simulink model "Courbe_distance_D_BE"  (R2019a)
settings: Solver=VariableStepAuto  StartTime=0.0  StopTime=6.283185307  MaxStep=0.001  RelTol=1e-6  SampleTimeConstraint=STIndependent

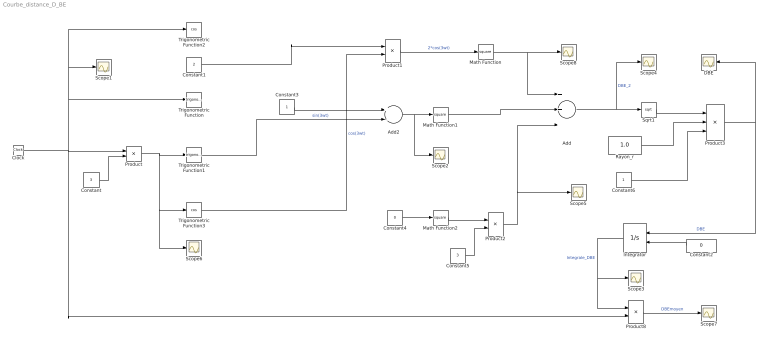
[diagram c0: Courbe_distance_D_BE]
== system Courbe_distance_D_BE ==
  Add : Sum  Inputs=+++
  Add2 : Sum  Inputs=+-
  Clock : Clock
  Constant : Constant  Value=3
  Constant1 : Constant  Value=2
  Constant2 : Constant  Value=0
  Constant3 : Constant
  Constant4 : Constant  Value=0
  Constant5 : Constant  Value=3
  Constant6 : Constant
  DBE : Scope
  Integrator : Integrator  InitialConditionSource=external
  Math Function : Math  Operator=square
  Math Function1 : Math  Operator=square
  Math Function2 : Math  Operator=square
  Product : Product
  Product1 : Product
  Product2 : Product
  Product3 : Product  Inputs=**/
  Product8 : Product  Inputs=*/
  Rayon_r : Constant  Value=1.0
  Scope{1..8} (8 alike) : Scope
  Sqrt1 : Sqrt
  Trigonometric Function : Trigonometry
  Trigonometric Function1 : Trigonometry
  Trigonometric Function2 : Trigonometry  Operator=cos
  Trigonometric Function3 : Trigonometry  Operator=cos
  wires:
  Product/1 -> Scope6/1, Trigonometric Function3/1, Trigonometric Function1/1
  Constant/1 -> Product/2
  Clock/1 -> Product8/2, Trigonometric Function/1, Trigonometric Function2/1, Scope1/1, Product/1
  Add2/1 -> Scope2/1, Math Function1/1
  Math Function/1 -> Scope8/1, Add/1
  Add/1 -> Sqrt1/1, Scope4/1  "DBE_2"
  Integrator/1 -> Product8/1, Scope3/1  "Integrale_DBE"
  Constant2/1 -> Integrator/2
  Product8/1 -> Scope7/1  "DBEmoyen"
  Trigonometric Function3/1 -> Product1/2  "cos(3wt)"
  Trigonometric Function1/1 -> Add2/2  "sin(3wt)"
  Constant5/1 -> Product2/2
  Product2/1 -> Add/3, Scope5/1
  Sqrt1/1 -> Product3/1
  Rayon_r/1 -> Product3/2
  Constant6/1 -> Product3/3
  Product3/1 -> Integrator/1, DBE/1  "DBE"
  Product1/1 -> Math Function/1  "2*cos(3wt)"
  Constant1/1 -> Product1/1
  Constant3/1 -> Add2/1
  Math Function1/1 -> Add/2
  Math Function2/1 -> Product2/1
  Constant4/1 -> Math Function2/1
